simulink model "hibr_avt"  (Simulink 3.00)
settings: Solver=ode45  StartTime=0.0  StopTime=100.0  RelTol=1e-3
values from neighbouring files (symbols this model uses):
  vx = 2/5    (= 0.4)    [Init.m]
  vy = 3/5    (= 0.6)    [Init.m]
  x0 = 5    [Init.m]    (also in RTSINH.M = cputime; RTSINH_f.M = cputime)
  y0 = 2    [Init.m]
libraries: simulink3 x1

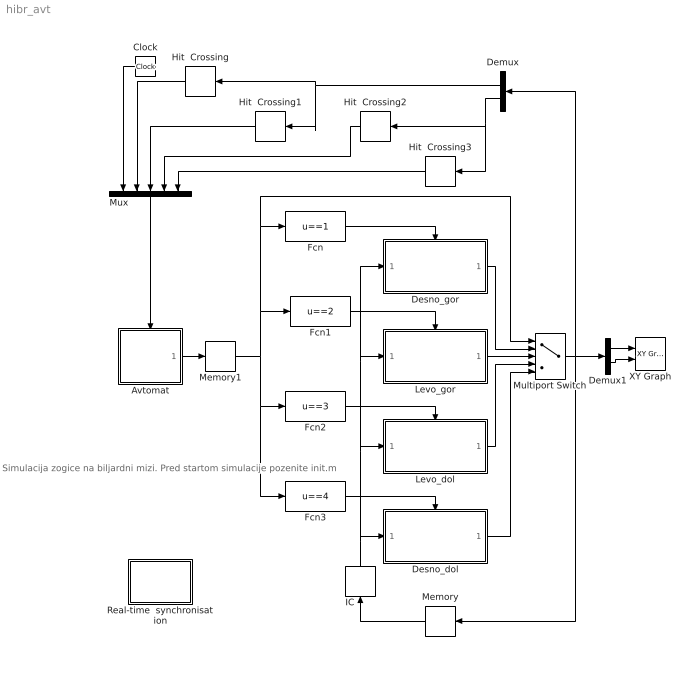
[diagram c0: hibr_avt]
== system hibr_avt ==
  note: Simulacija zogice na biljardni mizi. Pred startom simulacije pozenite init.m
  Avtomat : Stateflow chart
  Clock : Clock
  Demux : Demux  Orientation=left  Outputs=2
  Demux1 : Demux  Outputs=2
  Desno_dol : Subsystem
  Desno_gor : Subsystem
  Fcn : Fcn  Expr=u==1
  Fcn1 : Fcn  Expr=u==2
  Fcn2 : Fcn  Expr=u==3
  Fcn3 : Fcn  Expr=u==4
  Hit  Crossing : HitCross  Orientation=left  HitCrossingOffset=7  HitCrossingDirection=rising  ShowOutputPort=on
  Hit  Crossing1 : HitCross  Orientation=left  HitCrossingOffset=0  HitCrossingDirection=falling  ShowOutputPort=on
  Hit  Crossing2 : HitCross  Orientation=left  HitCrossingOffset=3  HitCrossingDirection=rising  ShowOutputPort=on
  Hit  Crossing3 : HitCross  Orientation=left  HitCrossingOffset=0  HitCrossingDirection=falling  ShowOutputPort=on
  IC : InitialCondition  Orientation=up  Value=[x0;y0]
  Levo_dol : Subsystem
  Levo_gor : Subsystem
  Memory : Memory  Orientation=left  X0=0  InheritSampleTime=off
  Memory1 : Memory  X0=1  InheritSampleTime=off
  Multiport Switch : MultiPortSwitch  Inputs=4
  Mux : Mux  Orientation=down  Inputs=5
  Real-time  synchronisation : Subsystem  mask(Real-time synchronisation){}
      mask help: Real-time synchronisation block
      mask init:
      | ts=@1;
  XY Graph : simulink3/Sinks/XY Graph  xmin=-1  xmax=8  ymin=-1  ymax=4  st=-1
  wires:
  Desno_gor/1("[x;y]") -> Multiport Switch/2
  Levo_gor/1("[x;y]") -> Multiport Switch/3
  Multiport Switch/1 -> Demux/1, Memory/1, Demux1/1
  Levo_dol/1("[x;y]") -> Multiport Switch/4
  Clock/1 -> Mux/1
  Hit  Crossing/1 -> Mux/2
  Hit  Crossing1/1 -> Mux/3
  Hit  Crossing2/1 -> Mux/4
  Fcn/1 -> Desno_gor/Enable
  Fcn2/1 -> Levo_dol/Enable
  Fcn3/1 -> Desno_dol/Enable
  Fcn1/1 -> Levo_gor/Enable
  Memory/1 -> IC/1
  Demux/1 -> Hit  Crossing1/1, Hit  Crossing/1
  Demux/2 -> Hit  Crossing2/1, Hit  Crossing3/1
  Memory1/1 -> Fcn1/1, Fcn/1, Multiport Switch/1, Fcn2/1, Fcn3/1
  IC/1 -> Desno_gor/1("[x0;y0]"), Levo_gor/1("[x0;y0]"), Levo_dol/1("[x0;y0]"), Desno_dol/1("[x0;y0]")
  Hit  Crossing3/1 -> Mux/5
  Desno_dol/1("[x;y]") -> Multiport Switch/5
  Mux/1 -> Avtomat/Trigger
  Avtomat/1(l) -> Memory1/1
  Demux1/1 -> XY Graph/1
  Demux1/2 -> XY Graph/2

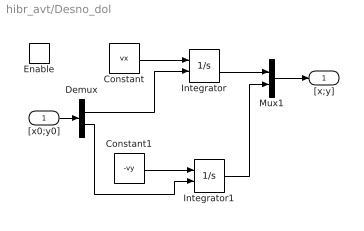
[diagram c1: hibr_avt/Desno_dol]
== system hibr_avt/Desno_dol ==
  "[x0;y0]" : Inport  Port=1  PortWidth=-1  SampleTime=-1  DataType=auto
  Enable : EnablePort  StatesWhenEnabling=reset
  Constant : Constant  Value=vx
  Constant1 : Constant  Value=-vy
  Demux : Demux  Outputs=2
  Integrator : Integrator  ExternalReset=none  InitialConditionSource=external  InitialCondition=0  LimitOutput=off  UpperSaturationLimit=inf  LowerSaturationLimit=-inf  ShowSaturationPort=off  ShowStatePort=off  AbsoluteTolerance=auto
  Integrator1 : Integrator  ExternalReset=none  InitialConditionSource=external  InitialCondition=0  LimitOutput=off  UpperSaturationLimit=inf  LowerSaturationLimit=-inf  ShowSaturationPort=off  ShowStatePort=off  AbsoluteTolerance=auto
  Mux1 : Mux  Inputs=2
  "[x;y]" : Outport  Port=1
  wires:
  Integrator1/1 -> Mux1/2
  Constant1/1 -> Integrator1/1
  Constant/1 -> Integrator/1
  Integrator/1 -> Mux1/1
  Mux1/1 -> "[x;y]"/1
  "[x0;y0]"/1 -> Demux/1
  Demux/1 -> Integrator/2
  Demux/2 -> Integrator1/2

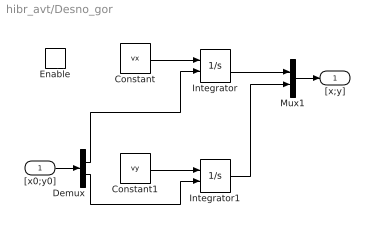
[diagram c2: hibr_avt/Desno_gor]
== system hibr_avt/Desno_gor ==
  "[x0;y0]" : Inport  Port=1  PortWidth=-1  SampleTime=-1  DataType=auto
  Enable : EnablePort  StatesWhenEnabling=reset
  Constant : Constant  Value=vx
  Constant1 : Constant  Value=vy
  Demux : Demux  Outputs=2
  Integrator : Integrator  ExternalReset=none  InitialConditionSource=external  InitialCondition=0  LimitOutput=off  UpperSaturationLimit=inf  LowerSaturationLimit=-inf  ShowSaturationPort=off  ShowStatePort=off  AbsoluteTolerance=auto
  Integrator1 : Integrator  ExternalReset=none  InitialConditionSource=external  InitialCondition=0  LimitOutput=off  UpperSaturationLimit=inf  LowerSaturationLimit=-inf  ShowSaturationPort=off  ShowStatePort=off  AbsoluteTolerance=auto
  Mux1 : Mux  Inputs=2
  "[x;y]" : Outport  Port=1
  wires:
  Constant/1 -> Integrator/1
  Constant1/1 -> Integrator1/1
  Integrator/1 -> Mux1/1
  Integrator1/1 -> Mux1/2
  Mux1/1 -> "[x;y]"/1
  "[x0;y0]"/1 -> Demux/1
  Demux/1 -> Integrator/2
  Demux/2 -> Integrator1/2

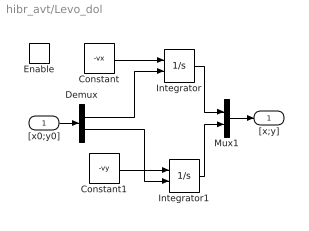
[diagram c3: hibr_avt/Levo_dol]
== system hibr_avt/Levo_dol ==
  "[x0;y0]" : Inport  Port=1  PortWidth=-1  SampleTime=-1  DataType=auto
  Enable : EnablePort  StatesWhenEnabling=reset
  Constant : Constant  Value=-vx
  Constant1 : Constant  Value=-vy
  Demux : Demux  Outputs=2
  Integrator : Integrator  ExternalReset=none  InitialConditionSource=external  InitialCondition=0  LimitOutput=off  UpperSaturationLimit=inf  LowerSaturationLimit=-inf  ShowSaturationPort=off  ShowStatePort=off  AbsoluteTolerance=auto
  Integrator1 : Integrator  ExternalReset=none  InitialConditionSource=external  InitialCondition=0  LimitOutput=off  UpperSaturationLimit=inf  LowerSaturationLimit=-inf  ShowSaturationPort=off  ShowStatePort=off  AbsoluteTolerance=auto
  Mux1 : Mux  Inputs=2
  "[x;y]" : Outport  Port=1
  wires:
  Constant/1 -> Integrator/1
  Constant1/1 -> Integrator1/1
  "[x0;y0]"/1 -> Demux/1
  Demux/1 -> Integrator/2
  Integrator/1 -> Mux1/1
  Mux1/1 -> "[x;y]"/1
  Integrator1/1 -> Mux1/2
  Demux/2 -> Integrator1/2

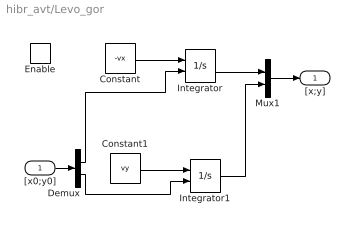
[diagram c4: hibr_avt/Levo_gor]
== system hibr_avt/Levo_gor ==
  "[x0;y0]" : Inport  Port=1  PortWidth=-1  SampleTime=-1  DataType=auto
  Enable : EnablePort  StatesWhenEnabling=reset
  Constant : Constant  Value=-vx
  Constant1 : Constant  Value=vy
  Demux : Demux  Outputs=2
  Integrator : Integrator  ExternalReset=none  InitialConditionSource=external  InitialCondition=0  LimitOutput=off  UpperSaturationLimit=inf  LowerSaturationLimit=-inf  ShowSaturationPort=off  ShowStatePort=off  AbsoluteTolerance=auto
  Integrator1 : Integrator  ExternalReset=none  InitialConditionSource=external  InitialCondition=0  LimitOutput=off  UpperSaturationLimit=inf  LowerSaturationLimit=-inf  ShowSaturationPort=off  ShowStatePort=off  AbsoluteTolerance=auto
  Mux1 : Mux  Inputs=2
  "[x;y]" : Outport  Port=1
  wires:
  Integrator1/1 -> Mux1/2
  Constant1/1 -> Integrator1/1
  Constant/1 -> Integrator/1
  "[x0;y0]"/1 -> Demux/1
  Integrator/1 -> Mux1/1
  Mux1/1 -> "[x;y]"/1
  Demux/1 -> Integrator/2
  Demux/2 -> Integrator1/2

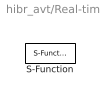
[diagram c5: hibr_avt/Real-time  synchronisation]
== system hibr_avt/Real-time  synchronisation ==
  S-Function : S-Function  FunctionName=rtsinh  Parameters=ts  PortCounts=[]  SFunctionModules=''

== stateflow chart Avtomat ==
  state desno_gor/l=1;
  state levo_gor/l=2;
  state levo_dol/l=3;
  state desno_dol/l=4;
  desno_gor/l=1; -> levo_gor/l=2; : x_l
  (default) -> desno_gor/l=1; : init
  levo_gor/l=2; -> desno_gor/l=1; : x_0
  desno_dol/l=4; -> desno_gor/l=1; : y_0
  desno_gor/l=1; -> desno_dol/l=4; : y_h
  levo_dol/l=3; -> levo_gor/l=2; : y_0
  levo_gor/l=2; -> levo_dol/l=3; : y_h
  desno_dol/l=4; -> levo_dol/l=3; : x_l
  levo_dol/l=3; -> desno_dol/l=4; : x_0
